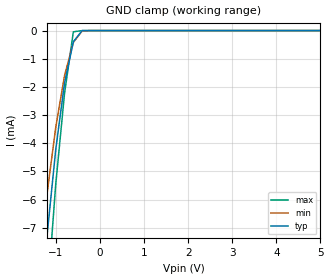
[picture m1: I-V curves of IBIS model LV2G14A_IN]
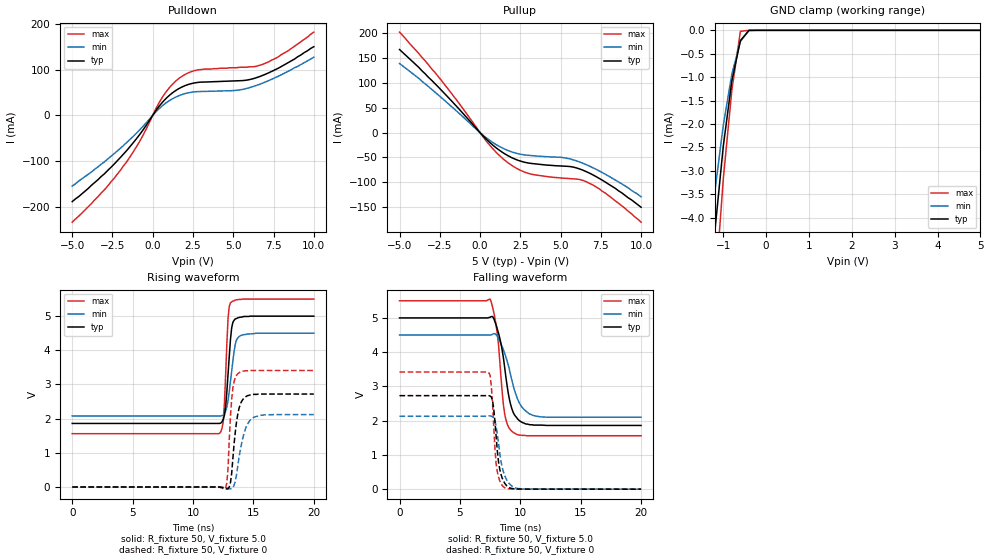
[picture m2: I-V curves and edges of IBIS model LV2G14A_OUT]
|/_/_/_/_/_/_/_/_/_/_/_/_/_/_/_/_/_/_/_/_/_/_/_/_/_/_/_/_/_/_/_/_/_/_/_/_/_/
|   Renesas Electronics Corp.
|   Multi Purpose Semiconductor Digital IC Design Group
|   IBIS Model of HD74LV2G14A
|   5.0V Triple Inverters with Schmitt-trigger Inputs,
|   SSOP-8(8pin) Package
|   History
|   V1.0   April   1, 2003   : First release.
|/_/_/_/_/_/_/_/_/_/_/_/_/_/_/_/_/_/_/_/_/_/_/_/_/_/_/_/_/_/_/_/_/_/_/_/_/_/
[IBIS Ver]   2.1
[Comment Char]  |_char
[File name]   l2g14s5.ibs
[File Rev]   1.1
[Date]   April 1, 2003
[Source]   Data created from SPICE simulations at
|   Renesas Electronics Corp.
[Notes]   RLC value of the Package is determined by assuming typical
|   conditions.
[Disclaimer]   This information is for modeling purposes only, and is not
|   guaranteed.
[Copyright]   Copyright 2003, Renesas Electronics Corp.,
|   All Rights Reserved.
|   Component  HD74LV2G14A
[Component]   HD74LV2G14A
[Manufacturer]  Renesas Electronics Corp.
[Package]
|   typ   min   max
R_pkg   0.099   0.095   0.102
L_pkg   1.740nH   1.680nH   1.790nH
C_pkg   0.140pF   0.140pF   0.150pF
[Pin]   signal_name   model_name   R_pin   L_pin   C_pin
1   1A   LV2G14A_IN   0.102   1.780nH   0.140pF
2   3Y   LV2G14A_OUT   0.097   1.710nH   0.150pF
3   2A   LV2G14A_IN   0.095   1.680nH   0.150pF
4   GND   GND   0.102   1.790nH   0.140pF
5   2Y   LV2G14A_OUT   0.101   1.790nH   0.140pF
6   3A   LV2G14A_IN   0.097   1.710nH   0.150pF
7   1Y   LV2G14A_OUT   0.097   1.710nH   0.150pF
8   VCC   POWER   0.102   1.790nH   0.140pF
| Models and submodels in the file (2): LV2G14A_IN (Input), LV2G14A_OUT (Output)
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|   Model  LV2G14A_IN
[Model]   LV2G14A_IN
Model_type  Input
Vinl = 1.50V
Vinh = 3.50V
| variable   typ   min   max
C_comp   2.85pF   2.75pF   2.95pF
| variable   typ   min   max
[Temperature range]   25   85   -40
| variable   typ   min   max
[Voltage range]   5.0V   4.5V   5.5V
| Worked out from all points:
|   GND clamp passes 1 mA (typ) near -0.68 V on its own axis
[GND Clamp]
|   Voltage   I(typ)   I(min)   I(max)
-5V       -128mA     -106mA     -157mA
-1.4V     -11mA      -8.74mA    -14.7mA
-1.2V     -7.33mA    -5.84mA    -9.68mA
-1V       -4.23mA    -3.44mA    -5.46mA
-800mV    -1.86mA    -1.6mA     -2.23mA
-600mV    -396uA     -418uA     -43uA
-400mV    -474nA     -10.9uA    -2.94nA
5V        10.1pA     35.9pA     10pA
|   Model  LV2G14A_OUT
[Model]   LV2G14A_OUT
Model_type  Output
Polarity   Inverting
Vmeas = 2.5V
| variable   typ   min   max
C_comp   6.85pF   6.75pF   6.95pF
| variable   typ   min   max
[Temperature range]   25   85   -40
| variable   typ   min   max
[Voltage range]   5.0V   4.5V   5.5V
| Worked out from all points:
|   slope of the pulldown table from 0 to 0.75 V, typ, clamps not added: 22 ohm
|   slope of the pullup table from 0 to 0.75 V, typ, clamps not added: 31.4 ohm
|   GND clamp passes 1 mA (typ) near -0.78 V on its own axis
|   rising waveform, R_fixture 50, V_fixture 5.0: 20-80 % time 384ps typ, 513ps min, 288ps max; typ from 1.86 V to 5 V
|   rising waveform, R_fixture 50, V_fixture 0: 20-80 % time 501ps typ, 709ps min, 332ps max; typ from 0 V to 2.72 V
|   falling waveform, R_fixture 50, V_fixture 5.0: 20-80 % time 864ps typ, 1.19ns min, 620ps max; typ from 5 V to 1.86 V
|   falling waveform, R_fixture 50, V_fixture 0: 20-80 % time 479ps typ, 623ps min, 366ps max; typ from 2.73 V to 0 V
[Pullup]
|   Voltage   I(typ)   I(min)   I(max)
-5V       167mA      139mA      202mA
-2.4V     85.2mA     70.3mA     105mA
200mV     -6.98mA    -5.55mA    -8.94mA
1V        -30.6mA    -24.1mA    -39.5mA
1.6V      -43.9mA    -34.1mA    -57.2mA
2.4V      -56.1mA    -42.7mA    -74mA
3.2V      -62mA      -46.2mA    -83.6mA
5.2V      -67.4mA    -50.4mA    -91.6mA
5.8V      -69.4mA    -54.8mA    -92.9mA
6.6V      -78.5mA    -64.5mA    -98.7mA
7.8V      -99.8mA    -84mA      -122mA
10V       -150mA     -129mA     -180mA
[Pulldown]
|   Voltage   I(typ)   I(min)   I(max)
-5V       -189mA     -155mA     -234mA
-3V       -128mA     -102mA     -163mA
-1.6V     -76.4mA    -59.1mA    -101mA
-800mV    -41.6mA    -31.5mA    -56.3mA
600mV     28.4mA     20.9mA     39.7mA
1V        42.6mA     31.4mA     59.1mA
1.6V      57.9mA     42.5mA     79.9mA
2.8V      71.9mA     51.8mA     99.3mA
5.2V      75.3mA     54.5mA     104mA
6.8V      86.9mA     70mA       111mA
8.4V      115mA      96.1mA     141mA
10V       150mA      127mA      182mA
[GND Clamp]
|   Voltage   I(typ)   I(min)   I(max)
-5V       -76.6mA    -64mA      -93.9mA
-1.4V     -6.55mA    -5.21mA    -8.67mA
-1.2V     -4.33mA    -3.47mA    -5.69mA
-1V       -2.48mA    -2.03mA    -3.18mA
-800mV    -1.08mA    -936uA     -1.28mA
-600mV    -219uA     -237uA     -20.5uA
-400mV    -248nA     -6.13uA    -1.4nA
5V        5.14pA     37.3pA     5pA
[Ramp]
| variable   typ   min   max
dV/dt_r   1.636/500.0p   1.275/713.3p   2.049/333.0p
dV/dt_f   1.882/864.4p   1.446/1.200n   2.363/619.6p
R_load = 50ohms
[Rising Waveform]
R_fixture = 50
V_fixture = 5.0
V_fixture_min = 4.5
V_fixture_max = 5.5
C_fixture = 0p
|   Time   V(typ)   V(min)   V(max)
0s        1.86V      2.08V      1.56V
12.2ns    1.86V      2.08V      1.57V
12.5ns    1.98V      2.11V      1.91V
12.7ns    2.35V      2.22V      3.28V
12.9ns    3.31V      2.54V      4.94V
13.1ns    4.32V      3.09V      5.39V
13.3ns    4.82V      3.69V      5.44V
13.5ns    4.92V      4.18V      5.47V
13.8ns    4.96V      4.4V       5.49V
20ns      5V         4.5V       5.5V
[Rising Waveform]
R_fixture = 50
V_fixture = 0
C_fixture = 0p
|   Time   V(typ)   V(min)   V(max)
0s        19.9nV     553nV      95.8nV
12.6ns    -32.6mV    -14.3mV    -63.6mV
12.8ns    -60.2mV    -28.6mV    121mV
12.9ns    -53.3mV    -38.6mV    550mV
13.1ns    132mV      -55.8mV    2.07V
13.3ns    836mV      -17.5mV    2.9V
13.6ns    1.9V       357mV      3.27V
14.2ns    2.59V      1.54V      3.39V
14.8ns    2.7V       1.98V      3.41V
20ns      2.72V      2.12V      3.41V
[Falling Waveform]
R_fixture = 50
V_fixture = 5.0
V_fixture_min = 4.5
V_fixture_max = 5.5
C_fixture = 0p
|   Time   V(typ)   V(min)   V(max)
0s        5V         4.5V       5.5V
7.5ns     5.02V      4.5V       5.55V
7.8ns     4.99V      4.54V      5.17V
8.1ns     4.67V      4.46V      4.53V
8.7ns     3.57V      3.97V      2.21V
9.2ns     2.47V      3.33V      1.73V
9.7ns     2.09V      2.7V       1.6V
10.3ns    1.93V      2.33V      1.57V
11.3ns    1.87V      2.13V      1.56V
20ns      1.86V      2.1V       1.56V
[Falling Waveform]
R_fixture = 50
V_fixture = 0
C_fixture = 0p
|   Time   V(typ)   V(min)   V(max)
0s        2.73V      2.13V      3.42V
7.4ns     2.73V      2.14V      3.4V
7.6ns     2.69V      2.13V      3.02V
7.8ns     2.35V      2.08V      1.85V
8ns       1.54V      1.84V      737mV
8.3ns     581mV      1.05V      243mV
8.7ns     179mV      405mV      42.5mV
9.2ns     29.4mV     121mV      7.49mV
9.9ns     4.6mV      15.9mV     708uV
20ns      -319nV     -1.91uV    -227nV
